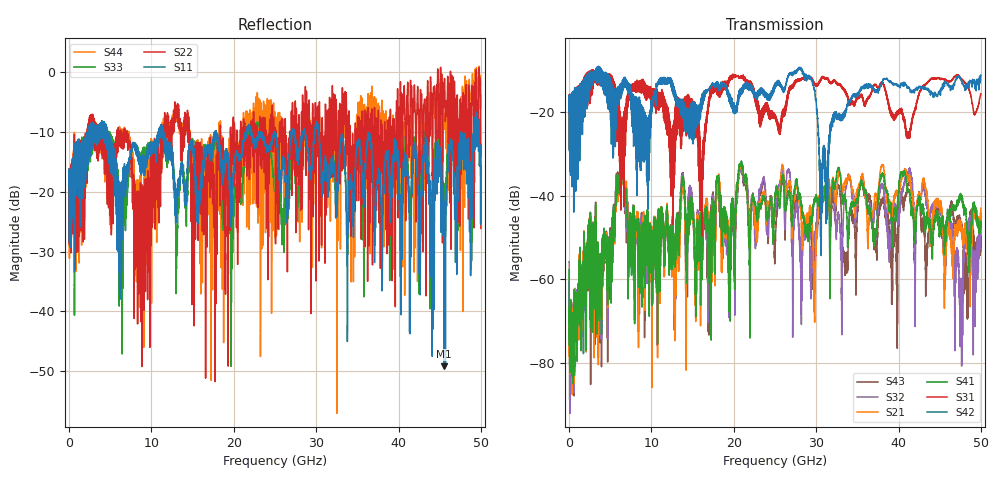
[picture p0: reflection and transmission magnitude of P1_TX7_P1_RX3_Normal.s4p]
!Keysight Technologies,N5225B,MY57041031,A.13.20.10
!Date: Friday, May 31, 2019 11:17:45
!Correction: S11(Full 4 Port(1,2,3,4))
!S12(Full 4 Port(1,2,3,4))
!S13(Full 4 Port(1,2,3,4))
!S14(Full 4 Port(1,2,3,4))
!S21(Full 4 Port(1,2,3,4))
!S22(Full 4 Port(1,2,3,4))
!S23(Full 4 Port(1,2,3,4))
!S24(Full 4 Port(1,2,3,4))
!S31(Full 4 Port(1,2,3,4))
!S32(Full 4 Port(1,2,3,4))
!S33(Full 4 Port(1,2,3,4))
!S34(Full 4 Port(1,2,3,4))
!S41(Full 4 Port(1,2,3,4))
!S42(Full 4 Port(1,2,3,4))
!S43(Full 4 Port(1,2,3,4))
!S44(Full 4 Port(1,2,3,4))
!S4P File: Measurements: <S11,S12,S13,S14>,
!<S21,S22,S23,S24>,
!<S31,S32,S33,S34>,
!<S41,S42,S43,S44>:
# Hz S  dB  R 50.0
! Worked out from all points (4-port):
!   5000 points, 10 MHz to 50 GHz, reference 50 ohm
!   strongest paths, dB at 10 MHz, 12.51 GHz, 25.01 GHz, 37.51 GHz, 50 GHz:
!     S42: -19.6, -14.4, -13.4, -15.1, -11.0
!     S31: -19.4, -39.4, -20.9, -14.0, -15.5
!     S41: -57.7, -51.0, -40.5, -41.0, -46.1
!     S21: -67.9, -52.6, -40.7, -40.6, -42.9
!     S32: -55.8, -50.2, -44.2, -43.8, -46.7
!     S43: -69.2, -50.3, -54.5, -46.8, -52.1
!   lowest |S11| = -49.2 dB at 45.52 GHz (marker M1), VSWR 1.01, Z = 49.7 + j0.205 ohm
!   |S11| at or under -10 dB: 4.613 GHz to 10.86 GHz (6.246 GHz wide, 80.7 % of centre); 11.46 GHz to 17.74 GHz (6.279 GHz wide, 43 % of centre); 30.28 GHz to 47.62 GHz (17.33 GHz wide, 44.5 % of centre)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
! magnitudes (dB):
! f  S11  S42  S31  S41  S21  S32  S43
! 10 MHz  -19.1  -19.6  -19.4  -57.7  -67.9  -55.8  -69.2
! 6.34 GHz  -19.2  -13.0  -37.8  -32.8  -33.9  -33.2  -32.3
! 9.95 GHz  -14.1  -18.5  -16.3  -51.0  -51.3  -51.2  -51.5
! 28.07 GHz  -11.9  -9.2  -12.0  -40.1  -42.6  -53.0  -51.8
! 30.63 GHz  -18.3  -40.5  -12.1  -43.6  -43.5  -43.1  -41.8
! 45.52 GHz  -49.2  -13.0  -12.0  -48.5  -55.6  -49.8  -47.8
! 50 GHz  -15.6  -11.0  -15.5  -46.1  -42.9  -46.7  -52.1
